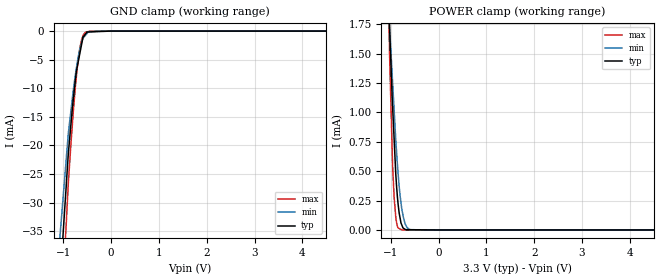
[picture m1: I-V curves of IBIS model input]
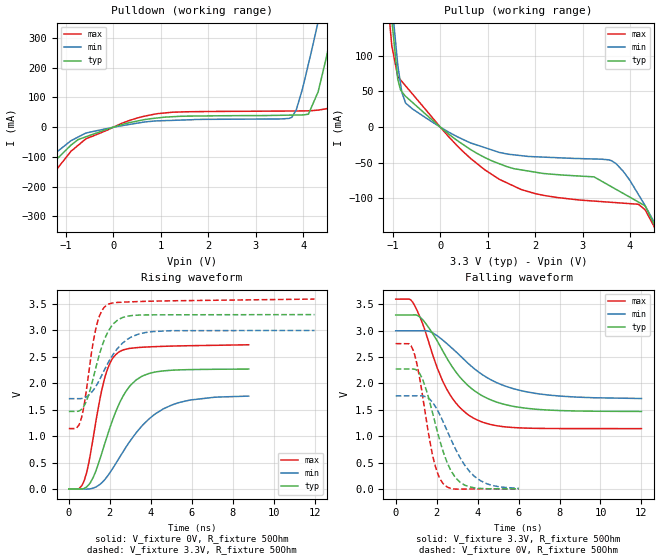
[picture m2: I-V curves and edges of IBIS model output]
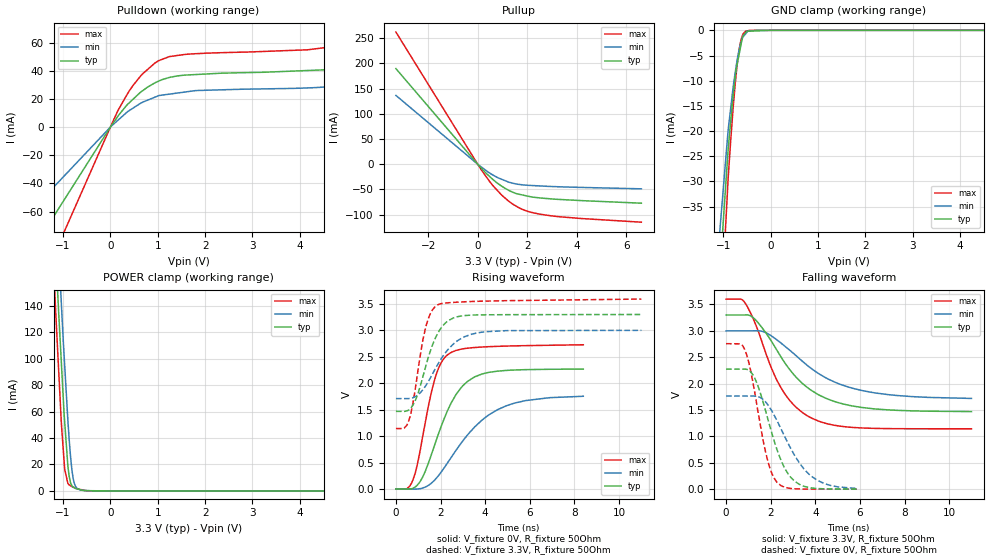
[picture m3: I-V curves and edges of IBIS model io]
|Texas Instruments Incorporated
| "SMART" 4-Wire Touch Screen Controller with Stereo DAC with HP Amplifier
| Marketing part#   Digital Voltage Range   Package-type   #pins
| TSC2102IDA   2.7V - 3.6V   TSSOP   32
| TSC2102IDAG4   2.7V - 3.6V   TSSOP   32
| TSC2102IDAR   2.7V - 3.6V   TSSOP   32
| TSC2102IDARG4   2.7V - 3.6V   TSSOP   32
[IBIS Ver]   3.2
[File name]   tsc2102.ibs
|SIMDE Ver   V3.0 - 201101 - RHL4 - Build 457
[File Rev]   1.1
[Date]   9/15/2011
[Source]
| Texas Instruments Incorporated.
| Analog-eLab Design Center, HPA
| 12500 TI Blvd
| Dallas, TX -75243
| e-mail: elab_scm_ibis@list.ti.com
[Notes]   Revision History:
| Rev 1.1: 9/15/2011
| - Updated C_comp values without Bondpad.
| Rev 1.0: 8/23/2011
| - Initial version of the model
| - Model generated from simulations in TISPICE
| - Model matched to SPICE simulation
| - C_comp although listed in numerical order of value are
|   obtained from varying PVT conditions. For PVT conditions for
|   each specific value refer the buffer description under
|   respective [Model]. IBIS model user is responsible for using
|   appropriate C_comp to simulate for Signal Integrity.
[Disclaimer]
| This model is designed as an aid for customers of Texas Instruments.
| TI and its licensors and suppliers make no warranties, either expressed
| or implied, with respect to this  model, including the warranties of
| merchantability or fitness for a particular purpose. The model is
| provided solely on an "as is" basis. The entire risk as to its quality
| and performance is with the customer.
[Copyright]
 (C) Copyright 2011 Texas Instruments Incorporated.All rights reserved.
|   TSC2102
[Component]   TSC2102
[Manufacturer]   TI
[Package]   |32 TSSOP   -  DA package
|   typ   min   max
R_pkg   0.20621   0.15801   0.27289
L_pkg   3.37560nH   2.40689nH   5.01067nH
C_pkg   0.79550pF   0.66567pF   0.94195pF
[Pin]  signal_name   model_name   R_pin   L_pin   C_pin
1   DIN   input   0.26799   4.84342nH  0.92339pF
2   NC   NC   0.12409   2.35955nH  0.76614pF
3   BCLK   io   0.21588   3.32515nH  0.80588pF
4   DVDD   power   0.15667   2.55370nH  0.84155pF
5   DVSS   gnd   0.14312   2.41927nH  0.80704pF
6   IOVDD   power   0.13500   2.38539nH  0.73508pF
7   MCLK   input   0.16852   2.52375nH  0.69134pF
8   SCLK   input   0.15877   2.41392nH  0.67038pF
9   MISO   output   0.15938   2.42311nH  0.69008pF
10   MOSI   input   0.16666   2.50863nH  0.68609pF
11   _SS   input   0.17706   2.63272nH  0.71647pF
12   _PINTDAV   output   0.19201   2.82730nH  0.77646pF
13   NC   NC   0.11134   1.66342nH  0.69912pF
14   NC   NC   0.10909   1.72904nH  0.69937pF
15   AUX   term   0.24310   4.20222nH  0.88234pF
16   VBAT2   term   0.26991   4.90180nH  0.93344pF
17   VBAT1   term   0.26263   4.81995nH  0.93117pF
18   VREF   term   0.23242   4.05017nH  0.88008pF
19   AVSS   gnd   0.15019   2.79631nH  0.85162pF
20   Y-   term   0.19482   2.96952nH  0.79400pF
21   X-   term   0.18396   2.75027nH  0.77804pF
22   Y+   term   0.17374   2.60830nH  0.71763pF
23   X+   term   0.16588   2.49631nH  0.68584pF
24   AVDD   power   0.11707   2.19794nH  0.69634pF
25   HPL   term   0.15801   2.40689nH  0.66567pF
26   DRVSS   gnd   0.12264   2.26194nH  0.73108pF
27   VGND   gnd   0.13246   2.42360nH  0.76410pF
28   DRVDD   power   0.14317   2.58784nH  0.82922pF
29   HPR   term   0.20226   3.17746nH  0.76570pF
30   _RESET   input   0.22150   3.69611nH  0.85132pF
31   LRCK   io   0.24293   4.29987nH  0.91818pF
32   _PWD   io   0.27289   5.01067nH  0.94195pF
33   THERMAL_PAD   NC   0.00008   0.00125nH  3.26032pF
[Pin Mapping]  pulldown_ref pullup_ref gnd_clamp_ref power_clamp_ref
1   GNDBUS3   PWRBUS2
2   NC   NC
3   GNDBUS1   PWRBUS2
4   NC   PWRBUS1
5   GNDBUS1   NC
6   NC   PWRBUS2
7   GNDBUS3   PWRBUS2
8   GNDBUS3   PWRBUS2
9   GNDBUS1   PWRBUS2
10   GNDBUS3   PWRBUS2
11   GNDBUS3   PWRBUS2
12   GNDBUS1   PWRBUS2
13   NC   NC
14   NC   NC
15   GNDBUS3   NC
16   GNDBUS3   PWRBUS3
17   GNDBUS3   PWRBUS3
18   GNDBUS3   PWRBUS3
19   GNDBUS2   NC
20   GNDBUS3   NC
21   GNDBUS3   NC
22   GNDBUS3   NC
23   GNDBUS3   NC
24   NC   PWRBUS3
25   GNDBUS3   PWRBUS4
26   GNDBUS3   NC
27   GNDBUS4   NC
28   NC   PWRBUS4
29   GNDBUS3   PWRBUS4
30   GNDBUS3   PWRBUS2
31   GNDBUS1   PWRBUS2
32   GNDBUS1   PWRBUS2
33   NC   NC
[Model] term
Model_type Terminator
C_comp   1.0e-20F  1.0e-20F  1.0e-20F
|   typ   min   max
[Voltage Range]   3.3V   3.0V   3.6V
[POWER Clamp Reference]   3.3V   3.0V   3.6V
[GND Clamp Reference]   0V   0V   0V
|Ambient Temperature   25   85   -40
|Junction Temperature
[Temperature Range]   25   85   -40
| Models and submodels in the file (4): input (Input), output (Output), io (I/O), term (Terminator)
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|   input Model
[Model]   input
Model_type   Input
Vinl = 0.99
Vinh = 2.31
|   typ   min   max
|   (nom PVT)   (fast PVT)   (slow PVT)
|C_comp from frequency sweep method (F=50MHz)
|Average
|C_comp   1.239e-12   1.232e-12   1.241e-12
|C_comp from LC tank measurement(L=1nH)
|Average
|Resonant Frequency(Hz)   5.090e+09   5.110e+09   5.089e+09
C_comp   9.787e-13   9.710e-13   9.790e-13
| Where nom  PVT is Nominal Process, 3.3V, 25C
|   Fast PVT is Strong Process,  3.6V, -40C
|   Slow PVT is Weak Process,   3V, 85C
[Model Spec]
|Subparameter   typ   min   max
Vinh   2.31   2.1   2.52
Vinl   0.99   0.9   1.08
[Voltage Range]   3.3   3   3.6
|Ambient Temperature   25   85   -40
|Junction Temperature
[Temperature Range]   25   85   -40
[Power Clamp Reference]   3.3   3   3.6
[GND Clamp Reference]   0   0   0
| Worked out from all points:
|   GND clamp passes 1 mA (typ) near -0.58 V on its own axis
|   POWER clamp passes 1 mA (typ) near -0.96 V on its own axis
[GND Clamp]
|   Voltage   I(typ)   I(min)   I(max)
-3.3V     -1.789A    -1.626A    -1.965A
-1.498V   -98.86mA   -79.77mA   -123.5mA
-897.6mV  -21.5mA    -17.99mA   -26.74mA
-792mV    -11.84mA   -10.3mA    -14.02mA
-726mV    -6.96mA    -6.356mA   -7.792mA
-702mV    -5.919mA   -5.132mA   -5.815mA
-658.8mV  -4.045mA   -3.308mA   -3.124mA
-622.8mV  -2.483mA   -2.109mA   -1.616mA
-590.7mV  -1.09mA    -1.282mA   -839.1uA
-532.8mV  -463.3uA   -676.9uA   -172.5uA
-285mV    -90.53uA   -1.014uA   -3.877uA
6.6V      0A         0A         0A
[POWER Clamp]
|   Voltage   I(typ)   I(min)   I(max)
-3.3V     32.16mA    22.45mA    56.05mA
-1.073V   2.242mA    2.096mA    2.407mA
-1.03V    1.742mA    1.743mA    1.532mA
-1.026V   1.703mA    1.714mA    1.468mA
-964.8mV  1.054mA    1.261mA    561.5uA
-932.4mV  774.8uA    1.021mA    280.4uA
-897.6mV  474.9uA    763.5uA    109.9uA
-861.3mV  271.9uA    544.7uA    29.15uA
-774mV    45.15uA    186.4uA    570.6nA
-699mV    4.775uA    49.29uA    19.85nA
-591mV    2.06uA     2.742uA    0A
6.6V      0A         0A         0A
|   output Model
[Model]   output
Model_type   Output
Polarity   Non-Inverting
Vmeas = 1.65
Vref = 1.65
Cref = 10pF
Rref = 50
|   typ   min   max
|   (nom PVT)   (fast PVT)   (slow PVT)
|C_comp from frequency sweep method (F=13MHz)
|C_comp   3.792e-12   3.384e-12   4.175e-12
|ON state : BUFFER OUTPUT TURNED HIGH
|C_comp   3.792e-12   3.384e-12   4.175e-12
|OFF state: BUFFER OUTPUT TURNED LOW
|C_comp   2.682e-12   2.597e-12   2.696e-12
|C_comp from LC tank measurement(L=1nH)
|Resonant Frequency(Hz)   4.140e+09   4.170e+09   4.070e+09
C_comp   1.479e-12   1.458e-12   1.531e-12
|ON state : BUFFER OUTPUT TURNED HIGH
|Resonant Frequency(Hz)   4.140e+09   4.170e+09   4.070e+09
|C_comp   1.479e-12   1.458e-12   1.531e-12
|OFF state: BUFFER OUTPUT TURNED LOW
|Resonant Frequency(Hz)   4.380e+09   4.390e+09   4.370e+09
|C_comp   1.322e-12   1.316e-12   1.328e-12
| Where nom  PVT is Nominal Process, 3.3V, 25C
|   Fast PVT is Strong Process,  3.6V, -40C
|   Slow PVT is Weak Process,   3V, 85C
[Voltage Range]   3.3   3   3.6
|Ambient Temperature   25   85   -40
|Junction Temperature
[Temperature Range]   25   85   -40
[Pullup Reference]   3.3   3   3.6
[Pulldown Reference]   0   0   0
[Power Clamp Reference]   3.3   3   3.6
[GND Clamp Reference]   0   0   0
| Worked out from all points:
|   slope of the pulldown table from 0 to 0.495 V, typ, clamps not added: 24.4 ohm
|   slope of the pullup table from 0 to 0.495 V, typ, clamps not added: 19.8 ohm
|   falling waveform, V_fixture 3.3V, R_fixture 50Ohm: 20-80 % time 2.12ns typ, 2.66ns min, 1.59ns max; typ from 3.3 V to 1.47 V
|   rising waveform, V_fixture 0V, R_fixture 50Ohm: 20-80 % time 1.32ns typ, 2.09ns min, 815ps max; typ from 0 V to 2.27 V
|   rising waveform, V_fixture 3.3V, R_fixture 50Ohm: 20-80 % time 851ps typ, 1.22ns min, 597ps max; typ from 1.47 V to 3.3 V
|   falling waveform, V_fixture 0V, R_fixture 50Ohm: 20-80 % time 1.02ns typ, 1.4ns min, 734ps max; typ from 2.27 V to 0 V
[Pulldown]
|   Voltage   I(typ)   I(min)   I(max)
-3.3V     -1.748A    -1.565A    -1.945A
-2.131V   -587.6mA   -459.7mA   -738.7mA
-1.947V   -412.8mA   -298.6mA   -557.7mA
-1.739V   -237.4mA   -174.9mA   -353.9mA
-1.505V   -156.9mA   -123.1mA   -204.3mA
-591mV    -33.04mA   -20.55mA   -40.6mA
939.6mV   31.11mA    21.1mA     45.54mA
3.753V    40.45mA    32.27mA    54.2mA
4.314V    118.1mA    353.3mA    57.23mA
4.662V    365.3mA    608mA      123.1mA
5.072V    676.5mA    916.8mA    425.6mA
6.6V      1.89A      2.099A     1.69A
[Pullup]
|   Voltage   I(typ)   I(min)   I(max)
-3.3V     1.913A     1.902A     1.946A
-1.267V   312.5mA    347.4mA    292mA
-1.022V   150.2mA    175.2mA    113.9mA
-897.6mV  67.44mA    87.36mA    71.24mA
-732mV    43.24mA    33.76mA    57.89mA
633.6mV   -31.28mA   -22.07mA   -43.6mA
1.706V    -59.96mA   -40.01mA   -87.56mA
3.612V    -83.75mA   -47.19mA   -105.5mA
4.183V    -105.3mA   -95.19mA   -108.5mA
4.508V    -136.5mA   -133.3mA   -139.8mA
4.74V     -174.6mA   -175.5mA   -181.8mA
6.6V      -1.764A    -1.852A    -1.671A
[Ramp]
R_load = 50
|   typ   min   max
dV/dt_r   1.36334/1.31672e-09   1.05841/2.1044e-09   1.64818/8.23212e-10
dV/dt_f   1.09866/2.11245e-09   0.771194/2.66396e-09   1.47398/1.58809e-09
[Falling Waveform]
V_fixture = 3.3V
V_fixture_min = 3V
V_fixture_max = 3.6V
R_fixture = 50Ohm
|   Time   V(typ)   V(min)   V(max)
0s        3.3V       3V         3.6V
838ps     3.301V     3V         3.538V
1.393ns   3.175V     3.002V     3.051V
1.996ns   2.828V     2.915V     2.33V
2.457ns   2.508V     2.77V      1.919V
3.1ns     2.138V     2.544V     1.557V
3.864ns   1.856V     2.272V     1.329V
5.196ns   1.615V     1.973V     1.183V
6.804ns   1.513V     1.813V     1.149V
12ns      1.469V     1.715V     1.143V
[Rising Waveform]
V_fixture = 0V
V_fixture_min = 0V
V_fixture_max = 0V
R_fixture = 50Ohm
|   Time   V(typ)   V(min)   V(max)
0s        1.286nV    6.942nV    793.1pV
501ps     -2.596mV   -15.48uV   7.116mV
759ps     11.89mV    -2.281mV   167.6mV
1.192ns   220.3mV    16.51mV    974.3mV
1.746ns   846.6mV    172.9mV    2.091V
2.066ns   1.227V     342.3mV    2.424V
2.441ns   1.598V     574.4mV    2.591V
3.315ns   2.071V     1.076V     2.675V
4.629ns   2.236V     1.519V     2.7V
8.785ns   2.269V     1.758V     2.729V
[Rising Waveform]
V_fixture = 3.3V
V_fixture_min = 3V
V_fixture_max = 3.6V
R_fixture = 50Ohm
|   Time   V(typ)   V(min)   V(max)
0s        1.468V     1.71V      1.143V
382ps     1.467V     1.71V      1.156V
578ps     1.495V     1.71V      1.294V
872ps     1.677V     1.747V     1.907V
1.335ns   2.318V     1.951V     3.061V
1.604ns   2.683V     2.148V     3.366V
1.909ns   2.972V     2.381V     3.493V
2.621ns   3.244V     2.76V      3.535V
3.703ns   3.294V     2.958V     3.55V
12ns      3.3V       3V         3.594V
[Falling Waveform]
V_fixture = 0V
V_fixture_min = 0V
V_fixture_max = 0V
R_fixture = 50Ohm
|   Time   V(typ)   V(min)   V(max)
0s        2.274V     1.765V     2.757V
653ps     2.274V     1.765V     2.754V
862ps     2.274V     1.765V     2.622V
1.268ns   2.117V     1.764V     1.877V
1.781ns   1.472V     1.65V      675.9mV
2.071ns   1.037V     1.47V      272.1mV
2.348ns   673.3mV    1.246V     86.13mV
2.947ns   200.8mV    736.2mV    -4.848mV
3.845ns   19.17mV    237.8mV    -907.6uV
6.02ns    92.97uV    8.124mV    111.8uV
|   io Model
[Model]   io
Model_type   I/O
Polarity   Non-Inverting
Enable   Active-Low
Vinl = 0.99
Vinh = 2.31
Vmeas = 1.65
Vref = 1.65
Cref = 10pF
Rref = 50
|   typ   min   max
|   (nom PVT)   (fast PVT)   (slow PVT)
|C_comp from frequency sweep method (F=13MHz)
|Average
|C_comp   2.863e-12   2.648e-12   3.065e-12
|ON state : BUFFER OUTPUT TURNED HIGH
|C_comp   4.084e-12   3.666e-12   4.474e-12
|OFF state: BUFFER IN HIGH IMPEDANCE
|C_comp   1.642e-12   1.629e-12   1.656e-12
|C_comp from LC tank measurement(L=1nH)
|Average
|Resonant Frequency(Hz)   4.310e+09   4.340e+09   4.270e+09
C_comp   1.373e-12   1.353e-12   1.400e-12
|ON state : BUFFER OUTPUT TURNED HIGH
|Resonant Frequency(Hz)   4.130e+09   4.170e+09   4.070e+09
|C_comp   1.487e-12   1.458e-12   1.531e-12
|OFF state: BUFFER IN HIGH IMPEDANCE
|Resonant Frequency(Hz)   4.490e+09   4.510e+09   4.470e+09
|C_comp   1.258e-12   1.247e-12   1.269e-12
| Where nom  PVT is Nominal Process, 3.3V, 25C
|   Fast PVT is Strong Process,  3.6V, -40C
|   Slow PVT is Weak Process,   3V, 85C
[Model Spec]
|Subparameter   typ   min   max
Vinh   2.31   2.1   2.52
Vinl   0.99   0.9   1.08
[Voltage Range]   3.3   3   3.6
|Ambient Temperature   25   85   -40
|Junction Temperature
[Temperature Range]   25   85   -40
[Pullup Reference]   3.3   3   3.6
[Pulldown Reference]   0   0   0
[Power Clamp Reference]   3.3   3   3.6
[GND Clamp Reference]   0   0   0
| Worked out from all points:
|   slope of the pulldown table from 0 to 0.495 V, typ, clamps not added: 24.3 ohm
|   slope of the pullup table from 0 to 0.495 V, typ, clamps not added: 19.8 ohm
|   GND clamp passes 1 mA (typ) near -0.57 V on its own axis
|   POWER clamp passes 1 mA (typ) near -0.64 V on its own axis
|   falling waveform, V_fixture 3.3V, R_fixture 50Ohm: 20-80 % time 2.13ns typ, 2.66ns min, 1.61ns max; typ from 3.3 V to 1.47 V
|   rising waveform, V_fixture 0V, R_fixture 50Ohm: 20-80 % time 1.32ns typ, 2.09ns min, 821ps max; typ from 0 V to 2.27 V
|   rising waveform, V_fixture 3.3V, R_fixture 50Ohm: 20-80 % time 852ps typ, 1.22ns min, 597ps max; typ from 1.47 V to 3.3 V
|   falling waveform, V_fixture 0V, R_fixture 50Ohm: 20-80 % time 1.02ns typ, 1.4ns min, 738ps max; typ from 2.27 V to 0.001 V
[Pulldown]
|   Voltage   I(typ)   I(min)   I(max)
-3.3V     -175mA     -117.5mA   -251.9mA
-3mV      -159.1uA   -106.9uA   -229uA
172.8mV   8.431mA    5.281mA    12.6mA
478.8mV   19.84mA    13.52mA    29.65mA
684mV     25.96mA    17.79mA    38.01mA
1.026V    32.84mA    22.46mA    47.35mA
1.591V    37.03mA    25.04mA    51.77mA
4.162V    40.27mA    27.89mA    54.99mA
5.141V    44.84mA    31.62mA    62.91mA
5.666V    52.29mA    36.11mA    74.45mA
6.154V    64.29mA    43.54mA    92.9mA
6.6V      80.98mA    50.36mA    118mA
[GND Clamp]
|   Voltage   I(typ)   I(min)   I(max)
-3.3V     -1.801A    -1.623A    -1.991A
-1.505V   -108.4mA   -89.16mA   -138.1mA
-897.6mV  -23.78mA   -19.9mA    -29.58mA
-792mV    -13.09mA   -11.39mA   -15.51mA
-726mV    -7.697mA   -7.027mA   -8.618mA
-702mV    -6.545mA   -5.674mA   -6.431mA
-658.8mV  -4.473mA   -3.656mA   -3.454mA
-622.8mV  -2.745mA   -2.331mA   -1.787mA
-590.7mV  -1.205mA   -1.416mA   -927.5uA
-532.8mV  -511.9uA   -747.8uA   -190.4uA
-285mV    -99.93uA   -1.117uA   -4.272uA
6.6V      0A         0A         0A
[Pullup]
|   Voltage   I(typ)   I(min)   I(max)
-3.3V     189.8mA    136.6mA    262.3mA
172.8mV   -9.547mA   -6.541mA   -13.21mA
633.6mV   -31.28mA   -22.07mA   -43.6mA
939.6mV   -42.69mA   -29.35mA   -59.94mA
1.246V    -51.68mA   -35.44mA   -73.23mA
1.554V    -58.32mA   -39.17mA   -83.32mA
1.886V    -61.91mA   -41.26mA   -91.35mA
2.473V    -66.64mA   -42.97mA   -98.8mA
4.162V    -72.11mA   -46mA      -107.7mA
6.6V      -77.32mA   -48.8mA    -115mA
[POWER Clamp]
|   Voltage   I(typ)   I(min)   I(max)
-3.3V     1.944A     1.96A      1.945A
-1.264V   264.5mA    312.7mA    221.5mA
-1.156V   182.6mA    229.5mA    136.4mA
-1.119V   155.1mA    201.5mA    110.6mA
-1.092V   135.7mA    182.1mA    91.77mA
-1.037V   98.42mA    143.3mA    52.64mA
-964.8mV  52.33mA    95.2mA     16.49mA
-871.2mV  11.3mA     39.84mA    4.607mA
-813mV    4.055mA    16.26mA    3.379mA
-745.8mV  1.975mA    4.331mA    2.257mA
-357mV    140uA      6.878uA    7.775uA
6.6V      0A         0A         0A
[Ramp]
R_load = 50
|   typ   min   max
dV/dt_r   1.36289/1.32113e-09   1.05776/2.11396e-09   1.64582/8.29156e-10
dV/dt_f   1.09777/2.12335e-09   0.768293/2.65758e-09   1.47376/1.61142e-09
[Falling Waveform]
V_fixture = 3.3V
V_fixture_min = 3V
V_fixture_max = 3.6V
R_fixture = 50Ohm
|   Time   V(typ)   V(min)   V(max)
0s        3.3V       3V         3.6V
832ps     3.301V     3V         3.542V
1.378ns   3.182V     3.002V     3.065V
2.006ns   2.822V     2.912V     2.323V
2.429ns   2.528V     2.779V     1.945V
3.044ns   2.167V     2.565V     1.592V
3.779ns   1.885V     2.3V       1.358V
4.848ns   1.663V     2.033V     1.211V
6.085ns   1.548V     1.87V      1.16V
11ns      1.47V      1.72V      1.144V
[Rising Waveform]
V_fixture = 0V
V_fixture_min = 0V
V_fixture_max = 0V
R_fixture = 50Ohm
|   Time   V(typ)   V(min)   V(max)
0s        1.291nV    7.116nV    793.1pV
500ps     -2.576mV   -11.96uV   6.658mV
763ps     12.58mV    -2.316mV   170.9mV
1.194ns   221.6mV    16.89mV    980.3mV
1.735ns   831.1mV    167.8mV    2.067V
2.308ns   1.476V     490.1mV    2.535V
3.228ns   2.04V      1.032V     2.663V
4.558ns   2.228V     1.5V       2.697V
5.823ns   2.257V     1.672V     2.711V
8.398ns   2.268V     1.753V     2.727V
[Rising Waveform]
V_fixture = 3.3V
V_fixture_min = 3V
V_fixture_max = 3.6V
R_fixture = 50Ohm
|   Time   V(typ)   V(min)   V(max)
0s        1.468V     1.71V      1.143V
382ps     1.467V     1.71V      1.155V
584ps     1.497V     1.71V      1.3V
924ps     1.73V      1.76V      2.052V
1.313ns   2.283V     1.937V     3.02V
1.552ns   2.618V     2.107V     3.325V
1.847ns   2.921V     2.335V     3.476V
2.553ns   3.229V     2.733V     3.527V
3.702ns   3.292V     2.956V     3.549V
11ns      3.3V       3V         3.591V
[Falling Waveform]
V_fixture = 0V
V_fixture_min = 0V
V_fixture_max = 0V
R_fixture = 50Ohm
|   Time   V(typ)   V(min)   V(max)
0s        2.274V     1.765V     2.757V
656ps     2.274V     1.765V     2.753V
862ps     2.274V     1.765V     2.621V
1.059ns   2.242V     1.765V     2.33V
1.323ns   2.068V     1.762V     1.746V
1.854ns   1.36V      1.611V     561.1mV
2.286ns   746.3mV    1.297V     129.4mV
2.89ns    230.4mV    778.6mV    14.6mV
3.836ns   23.37mV    241.9mV    1.814mV
5.906ns   1.162mV    12.33mV    482.9uV
